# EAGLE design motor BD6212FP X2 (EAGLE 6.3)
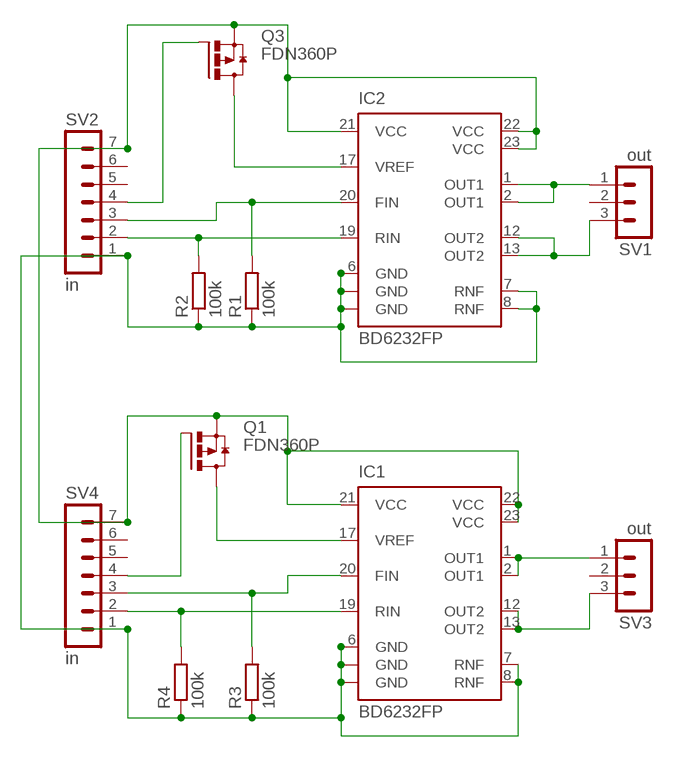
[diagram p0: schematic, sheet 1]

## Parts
IC1  BD6232FP  [HSOP25]
IC2  BD6232FP  [HSOP25]
Q1  FDN360P  [SUPER-SOT3]
Q3  FDN360P  [SUPER-SOT3]
R1  100k  R-EU_0204/7  [0204/7]
R2  100k  R-EU_0204/7  [0204/7]
R3  100k  R-EU_0204/7  [0204/7]
R4  100k  R-EU_0204/7  [0204/7]
SV1  out  MA03-1  [MA03-1]
SV2  in  MA07-1  [MA07-1]
SV3  out  MA03-1  [MA03-1]
SV4  in  MA07-1  [MA07-1]

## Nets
N$1: IC1.21(VCC) IC1.22(VCC) IC1.23(VCC) IC2.21(VCC) IC2.22(VCC) IC2.23(VCC) Q1.2(S) Q3.2(S) SV2.7 SV4.7
N$2: IC1.6(GND) IC1.7(RNF) IC1.8(RNF) IC1.GND@1(GND) IC1.GND@2(GND) IC2.6(GND) IC2.7(RNF) IC2.8(RNF) IC2.GND@1(GND) IC2.GND@2(GND) R1.1 R2.1 R3.1 R4.1 SV2.1 SV4.1
N$3: Q3.1(G) SV2.4
N$4: IC2.20(FIN) R1.2 SV2.3
N$5: IC2.19(RIN) R2.2 SV2.2
N$7: IC2.17(VREF) Q3.3(D)
N$8: IC2.1(OUT1) IC2.2(OUT1) SV1.1
N$9: IC2.12(OUT2) IC2.13(OUT2) SV1.3
N$11: IC1.19(RIN) R4.2 SV4.2
N$12: IC1.20(FIN) R3.2 SV4.3
N$13: IC1.17(VREF) Q1.3(D)
N$14: Q1.1(G) SV4.4
N$17: IC1.1(OUT1) IC1.2(OUT1) SV3.1
N$18: IC1.12(OUT2) IC1.13(OUT2) SV3.3
Unconnected: SV1.2 SV2.5 SV2.6 SV3.2 SV4.5 SV4.6

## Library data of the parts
IC1 IC2 = rohm:BD6232FP: H-bridge driver for brush motors Source: http://www.rohm.com/products/databook/motor/pdf/bd623x_series-e.pdf
Q1 Q3 = transistor-power:FDN360P: Single P-Channel, PowerTrench (R) MOSFET Source: http://www.fairchildsemi.com/ds/FD/FDN360P.pdf
R1-R4 = rcl:R-EU_: RESISTOR, European symbol
SV1 SV3 = con-lstb:MA03-1: PIN HEADER
SV2 SV4 = con-lstb:MA07-1: PIN HEADER

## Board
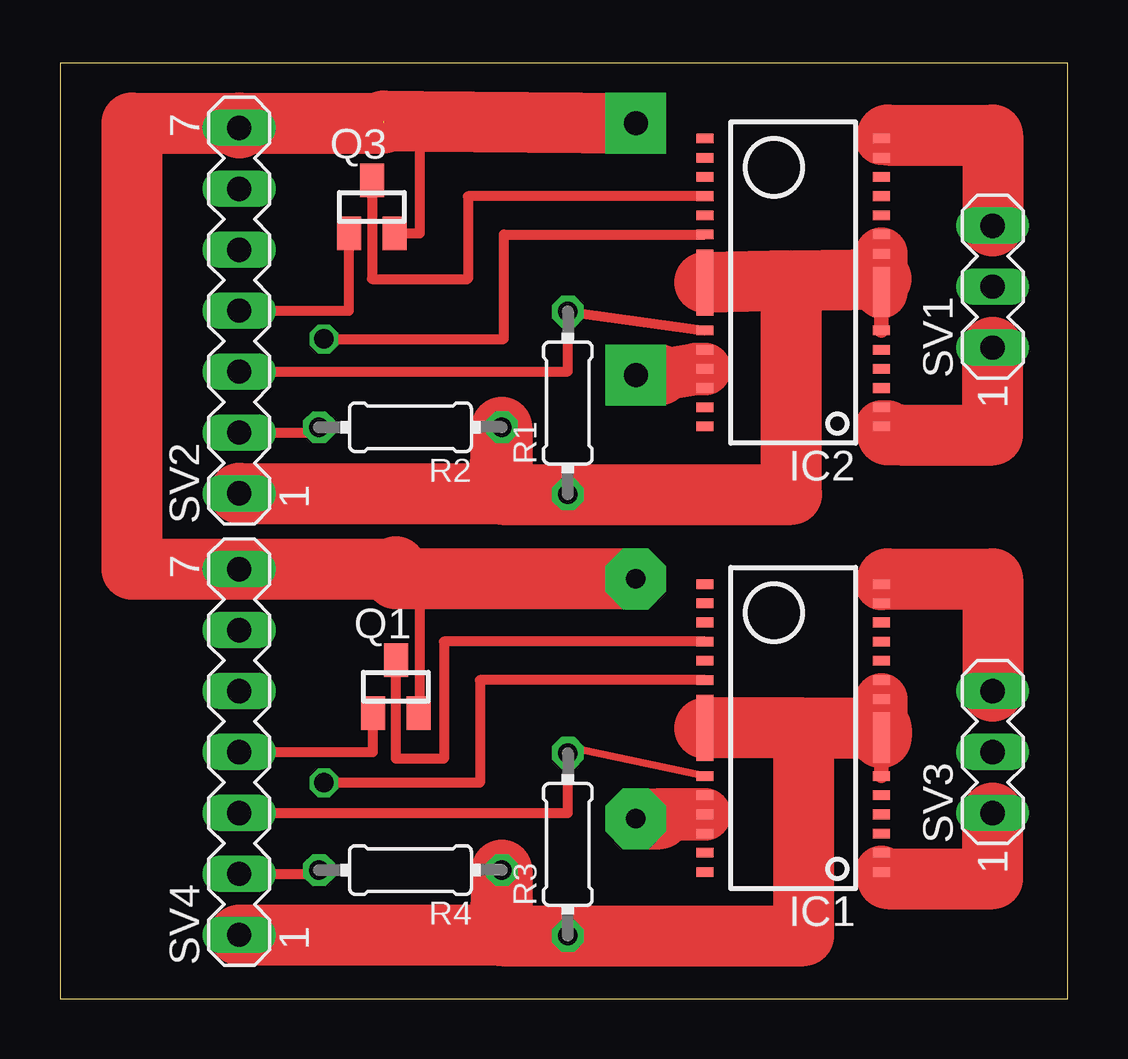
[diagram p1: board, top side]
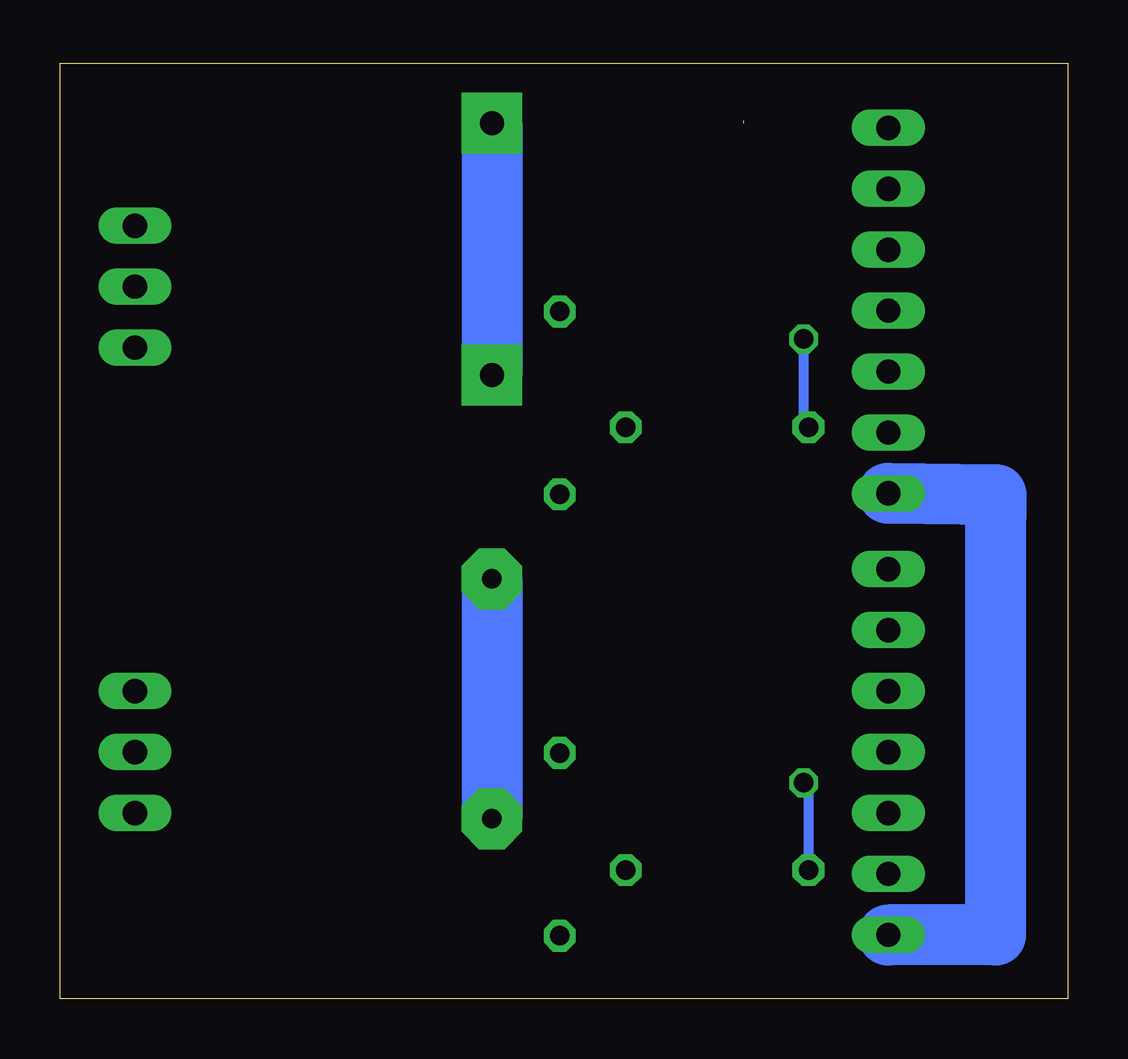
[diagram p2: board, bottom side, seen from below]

Size 42 x 39 mm. Coordinates in mm from the lower left corner, seen from the top.
Outline: 0,0 42,0 42,39 0,39 0,0
Copper layers (1*16): Top 0.035mm / dielectric 1.5mm / Bottom 0.035mm
Design rules "default": minimum track width 10mil, minimum drill 24mil, track to track 8mil, track to pad 8mil, pad to pad 8mil, via to via 8mil, smd to smd 8mil, copper to edge 40mil, drill to drill 8mil, minimum pad ring 10mil, minimum via ring 8mil, stop-mask expansion 4mil, vias tented up to drill 0mil, thermal gap 10mil

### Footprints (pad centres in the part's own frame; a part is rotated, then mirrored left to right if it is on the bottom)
HSOP25 = smd 0.4 x 0.7: 1 -6,-3.675; 2 -5.2,-3.675; 3 -4.4,-3.675; 4 -3.6,-3.675; 5 -2.8,-3.675; 6 -2,-3.675; 7 1.2,-3.675; 8 2,-3.675; 9 2.8,-3.675; 10 3.6,-3.675; 11 4.4,-3.675; 12 5.2,-3.675; 13 6,-3.675; 14 6,3.675; 15 5.2,3.675; 16 4.4,3.675; 17 3.6,3.675; 18 2.8,3.675; 19 2,3.675; 20 -2,3.675; 21 -2.8,3.675; 22 -3.6,3.675; 23 -4.4,3.675; 24 -5.2,3.675; 25 -6,3.675 | smd 2.1 x 0.7: GND@1 -0.4,-3.675 | smd 2.75 x 0.7: GND@2 0,3.675
SUPER-SOT3 = smd 1 x 1.4: 1 -0.95,-1.1; 2 0.95,-1.1; 3 0,1.1
0204/7 = drill 0.813 octagon: 1 -3.81,0; 2 3.81,0
MA03-1 = drill 1.016 long: 1 -2.54,0; 2 0,0; 3 2.54,0
MA07-1 = drill 1.016 long: 1 -7.62,0; 2 -5.08,0; 3 -2.54,0; 4 0,0; 5 2.54,0; 6 5.08,0; 7 7.62,0

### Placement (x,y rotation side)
IC1  30.56,11.28 90 top
IC2  30.56,29.85 90 top
Q1  14,13 0 top
Q3  13,33 0 top
R1  21.17,24.83 90 top
R2  14.61,23.82 180 top
R3  21.17,6.43 90 top
R4  14.61,5.36 180 top
SV1  38.88,29.68 90 top
SV2  7.47,28.68 90 top
SV3  38.88,10.28 90 top
SV4  7.47,10.28 90 top

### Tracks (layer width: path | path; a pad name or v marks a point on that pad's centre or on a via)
N$1  (via drill 0.8 pad 2.54, 1 pad 2.54)  (1 unrouted)
  Top 0.406: IC1.21 IC1.22 IC1.23 | IC2.21 IC2.22 IC2.23 | Q3.2 15.01,31.9 15.01,36.58 | Q1.2 15,11.9 15,18 14,18 13.59,18 13.59,17.9
  Top 2.184: IC2.22 26.5,26.25 25,26 | IC1.22 25,7.68 25,7.5
  Top 2.54: 13.5,36.59 15.01,36.58 v24,36.5 | v24,26 25,26 | 7.47,36.5 3,36.5 3,17.9 SV4.7 13.59,17.9 | 7.47,36.5 13.5,36.5 | 7.47,36.5 SV2.7 | v24,7.5 25,7.5 | v24,17.5 14,17.5 14,18
  Bottom 2.54: v24,36.5 v24,26 | v24,17.5 v24,7.5
N$2
  Top 0.406: IC2.7 IC2.8 | IC1.7 IC1.8
  Top 0.61: IC2.GND@1 IC2.6 | IC1.GND@1 IC1.6
  Top 2.184: IC2.GND@1 34.23,30 IC2.7 | IC1.GND@1 IC1.7
  Top 2.54: SV2.1 18.32,21.06 R2.1 18.42,21.02 R1.1 30.49,21.02 30.49,29.92 | SV4.1 18.36,2.66 R4.1 | R4.1 18.36,2.62 | 31,11.28 IC1.GND@2 | 31,11.28 34.23,11.28 IC1.GND@1 | 31,11.28 31,2.62 R3.1 18.42,2.62 R4.1 | 30.49,29.92 IC2.GND@2 | 30.49,29.92 34.23,30
  Bottom 2.54: SV4.1 3,2.66 3,19 2.97,21 SV2.1
N$3
  Top 0.406: SV2.4 12.05,28.68 Q3.1
N$4
  Top 0.406: SV2.3 21.17,26.14 R1.2 IC2.20
N$5  (via drill 0.8 pad 0.61)
  Top 0.406: SV2.2 10.4,23.6 R2.2 | IC2.19 18.5,31.85 18.5,28 18.5,27.5 v11,27.5
  Bottom 0.406: R2.2 11,23.82 v11,27.5
N$7
  Top 0.406: Q3.3 13,30 17,30 17,33.45 IC2.17
N$8
  Top 0.406: IC2.2 35,23.5
  Top 2.184: IC2.1 34.5,23.85 34.5,23.5
  Top 2.54: 34.5,23.5 35,23.5 38.88,23.5 SV1.1
N$9
  Top 0.406: IC2.13 IC2.12
  Top 2.184: IC2.13 34.5,35.85 34.5,36
  Top 2.54: 34.5,36 38.88,36 SV1.3
N$11  (via drill 0.8)
  Top 0.406: SV4.2 10.8,5.2 R4.2 | IC1.19 17.5,13.28 17.5,9 v11,9
  Bottom 0.406: v11,9 10.8,9 R4.2
N$12
  Top 0.305: IC1.20 21.17,10.5 R3.2
  Top 0.406: SV4.3 21.17,7.74 R3.2
N$13
  Top 0.406: IC1.17 16,14.88 16,10 14,10 Q1.3
N$14
  Top 0.406: SV4.4 13.05,10.28 Q1.1
N$17
  Top 0.406: IC1.2 IC1.1
  Top 2.184: 34.5,5 IC1.1
  Top 2.54: 34.5,5 38.88,5 SV3.1
N$18
  Top 0.406: IC1.12 IC1.13
  Top 2.184: IC1.13 34.5,17.5
  Top 2.54: 34.5,17.5 38.88,17.5 SV3.3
